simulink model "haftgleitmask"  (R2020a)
settings: Solver=ode45  StartTime=0.0  StopTime=3.5  MaxStep=0.01  RelTol=1e-6  AbsTol=1e-6

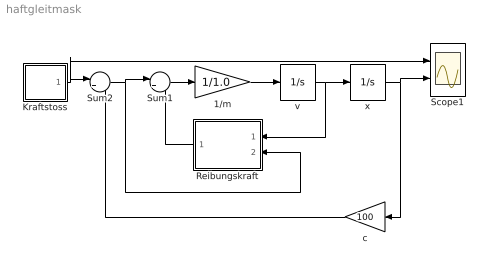
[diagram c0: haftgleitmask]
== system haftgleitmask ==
  note: .
  1/m : Gain  Gain=1/1.0  SaturateOnIntegerOverflow=on
  Kraftstoss : Subsystem  mask(Kraftstoss){tS=1.5, dt=0.1, Fmax=310}
      mask prompts: tS "Startzeit"; dt "Dauer"; Fmax "Staerke"
      mask help: Gibt einen Kraftstoss in Form eines Rechteckimpulses aus.
  Reibungskraft : Subsystem  mask(Reibungskraft){mug=0.8, muh=1.6, FN=50}
      mask prompts: mug "Gleitreibungskoeffizient"; muh "Haftreibungskoeffizient"; FN "Normalkraft"
      mask help: Berechnet die Reibungskraft fuer Haft- und Gleitreibung. Eingaenge: Geschwindigkeit, aeussere Kraft.
  Scope1 : Scope  NumInputPorts=2
  Sum1 : Sum  Inputs=|++  InputSameDT=on  SaturateOnIntegerOverflow=on
  Sum2 : Sum  Inputs=|+-  InputSameDT=on  SaturateOnIntegerOverflow=on
  c : Gain  Gain=100  SaturateOnIntegerOverflow=on
  v : Integrator
  x : Integrator  InitialCondition=3.5  UpperSaturationLimit=100  LowerSaturationLimit=-100
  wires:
  x/1 -> c/1, Scope1/2
  Sum1/1 -> 1/m/1
  v/1 -> x/1, Reibungskraft/1(v)
  1/m/1 -> v/1
  Reibungskraft/1(FR) -> Sum1/2
  c/1 -> Sum2/2
  Kraftstoss/1(Fext) -> Sum2/1, Scope1/1
  Sum2/1 -> Sum1/1, Reibungskraft/2(Fext)

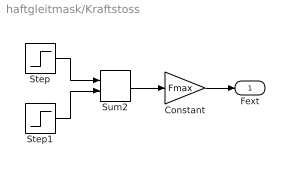
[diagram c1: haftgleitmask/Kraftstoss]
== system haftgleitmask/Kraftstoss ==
  Constant : Gain  Gain=Fmax  SaturateOnIntegerOverflow=on
  Step : Step  Time=tS  SampleTime=0
  Step1 : Step  Time=tS+dt  After=-1  SampleTime=0
  Sum2 : Sum  InputSameDT=on  SaturateOnIntegerOverflow=on
  Fext : Outport
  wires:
  Sum2/1 -> Constant/1
  Step/1 -> Sum2/1
  Step1/1 -> Sum2/2
  Constant/1 -> Fext/1

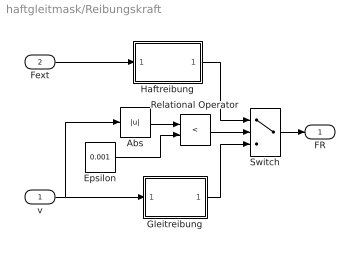
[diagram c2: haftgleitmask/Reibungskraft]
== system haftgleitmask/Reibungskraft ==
  v : Inport
  Fext : Inport  Port=2
  Abs : Abs
  Epsilon : Constant  Value=0.001
  Gleitreibung : Subsystem
  Haftreibung : Subsystem
  Relational Operator : RelationalOperator  Operator=<
  Switch : Switch  Threshold=0.5
  FR : Outport
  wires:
  Relational Operator/1 -> Switch/2
  Gleitreibung/1(Fg) -> Switch/3
  Haftreibung/1(Fh) -> Switch/1
  Epsilon/1 -> Relational Operator/2
  Abs/1 -> Relational Operator/1
  v/1 -> Abs/1, Gleitreibung/1(v)
  Fext/1 -> Haftreibung/1(Fext)
  Switch/1 -> FR/1

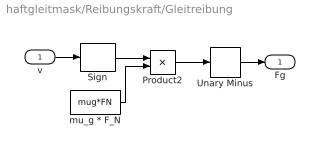
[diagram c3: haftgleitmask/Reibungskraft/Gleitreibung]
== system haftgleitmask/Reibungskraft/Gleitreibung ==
  v : Inport
  Product2 : Product  InputSameDT=on  SaturateOnIntegerOverflow=on
  Sign : Signum
  Unary Minus : UnaryMinus
  mu_g * F_N : Constant  Value=mug*FN
  Fg : Outport
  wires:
  Unary Minus/1 -> Fg/1
  Product2/1 -> Unary Minus/1
  v/1 -> Sign/1
  Sign/1 -> Product2/1
  mu_g * F_N/1 -> Product2/2

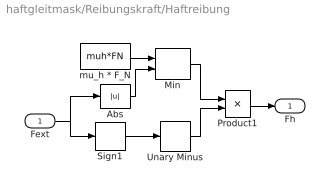
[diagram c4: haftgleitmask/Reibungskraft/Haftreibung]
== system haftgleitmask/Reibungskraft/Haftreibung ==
  Fext : Inport
  Abs : Abs
  Min : MinMax  Inputs=2  InputSameDT=on  SaturateOnIntegerOverflow=on
  Product1 : Product  InputSameDT=on  SaturateOnIntegerOverflow=on
  Sign1 : Signum
  Unary Minus : UnaryMinus
  mu_h * F_N : Constant  Value=muh*FN
  Fh : Outport
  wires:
  Unary Minus/1 -> Product1/2
  Sign1/1 -> Unary Minus/1
  Product1/1 -> Fh/1
  Fext/1 -> Sign1/1, Abs/1
  Min/1 -> Product1/1
  mu_h * F_N/1 -> Min/1
  Abs/1 -> Min/2
